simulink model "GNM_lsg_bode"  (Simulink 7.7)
settings: Solver=ode45  StartTime=0.0  StopTime=0.2  FixedStep=0.005  RelTol=1e-3
InitFcn:
  | GNM_lsg_ini
StopFcn:
  | GNMbode
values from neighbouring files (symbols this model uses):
  CE = 240.02    [GNM_lsg_ini.m]
  CM = CE/2/pi    (= 38.2003694409)    [GNM_lsg_ini.m]
  Fpwm = 5000    [GNM_lsg_ini.m]
  J = 0.012    [GNM_lsg_ini.m]
  LA = 0.004    [GNM_lsg_ini.m]
  psi = 0.04    [GNM_lsg_ini.m]
  RA = 0.25    [GNM_lsg_ini.m]
  Umax = 200    [GNM_lsg_ini.m]
libraries: simulink x3

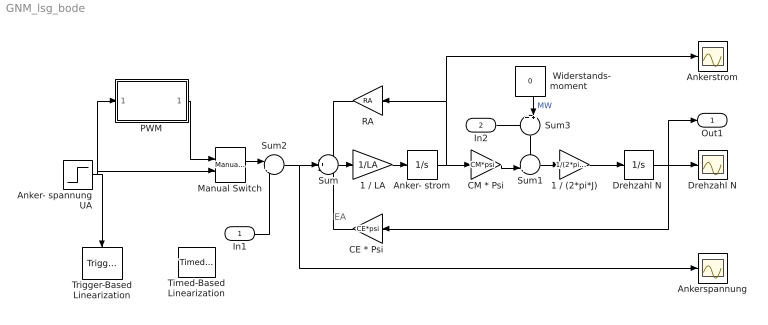
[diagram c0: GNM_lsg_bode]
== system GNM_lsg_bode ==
  note: EA
  In1 : Inport
  In2 : Inport  Port=2
  " Widerstands-  moment" : Constant  Value=0
  1 / (2*pi*J) : Gain  Gain=1/(2*pi*J)
  1 / LA : Gain  Gain=1/LA
  Anker- spannung UA : Step  Time=0.05  After=50  SampleTime=0
  Anker- strom : Integrator
  Ankerspannung : Scope
  Ankerstrom : Scope
  "CE * Psi " : Gain  Gain=CE*psi
  CM * Psi : Gain  Gain=CM*psi
  Drehzahl N : Scope
  "Drehzahl N " : Integrator
  Manual Switch : simulink/Signal Routing/Manual Switch  SystemSampleTime=-1  sw=0  action=0  varsize=off
  PWM : Subsystem
  RA : Gain  Gain=RA
  Sum : Sum  Inputs=-+-
  Sum1 : Sum  Inputs=-+|
  Sum2 : Sum  Inputs=|++
  Sum3 : Sum  Inputs=++|
  Timed-Based Linearization : simulink/Model-Wide Utilities/Timed-Based Linearization  SystemSampleTime=-1  LinearizationTime=0.1  SampleTime=0
  Trigger-Based Linearization : simulink/Model-Wide Utilities/Trigger-Based Linearization  SystemSampleTime=-1  TriggerType=rising  SampleTime=0
  Out1 : Outport
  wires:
  PWM/1(UAist) -> Manual Switch/1
  Anker- spannung UA/1 -> PWM/1(UAsoll), Manual Switch/2, Trigger-Based Linearization/Trigger
  In1/1 -> Sum2/2
  Manual Switch/1 -> Sum2/1
  RA/1 -> Sum/1
  Anker- strom/1 -> CM * Psi/1, RA/1, Ankerstrom/1
  Sum/1 -> 1 / LA/1
  1 / LA/1 -> Anker- strom/1
  CM * Psi/1 -> Sum1/2
  Sum1/1 -> 1 / (2*pi*J)/1
  1 / (2*pi*J)/1 -> "Drehzahl N "/1
  "CE * Psi "/1 -> Sum/3
  "Drehzahl N "/1 -> "CE * Psi "/1, Drehzahl N/1, Out1/1
  Sum2/1 -> Sum/2, Ankerspannung/1
  Sum3/1 -> Sum1/1
  In2/1 -> Sum3/1
  " Widerstands-  moment"/1 -> Sum3/2  "MW"

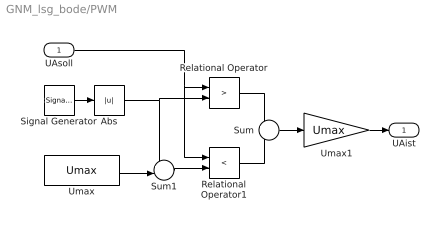
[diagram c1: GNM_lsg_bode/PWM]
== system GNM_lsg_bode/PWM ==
  UAsoll : Inport
  Abs : Abs
  Relational Operator : RelationalOperator  Operator=>
  Relational Operator1 : RelationalOperator  Operator=<
  Signal Generator : SignalGenerator  WaveForm=sawtooth  Amplitude=Umax  Frequency=Fpwm
  Sum : Sum  Inputs=+-
  Sum1 : Sum  Inputs=+-|
  Umax : Constant  Value=Umax
  Umax1 : Gain  Gain=Umax
  UAist : Outport  InitialOutput=0
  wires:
  Sum/1 -> Umax1/1
  Umax1/1 -> UAist/1
  Relational Operator1/1 -> Sum/2
  Relational Operator/1 -> Sum/1
  Umax/1 -> Sum1/2
  Abs/1 -> Sum1/1, Relational Operator/2
  UAsoll/1 -> Relational Operator/1, Relational Operator1/1
  Sum1/1 -> Relational Operator1/2
  Signal Generator/1 -> Abs/1
